|Texas Instruments Incorporated
|Reference-Less PCIe Gen 1-6 Compliant Programmable BAW Clock Generator
| Marketing Part # : LMK3H210X
| Digital Voltage Range : 1.8V, 2.5V, 3.3V
| Package-type: RER
| #pins/pkg drawing : 40/24-pin VQFN
[IBIS Ver] 4.1
[File name] lmk3h210x.ibs
[File Rev] 1.0
[Date] 06/26/2025
[Source]
| Texas Instruments Incorporated.
| 12500 TI Blvd
| Dallas, TX -75243
[Notes] Revision History:
| Rev 1.0: 6/26/2025
| - Initial version of the model
| - Model generated from simulations in TISPICE/SPECTRE
| - C_comp although listed in numerical order of value are
| obtained from varying PVT conditions. For PVT conditions for
| each specific value refer the buffer description under
| respective [Model]. IBIS model user is responsible for using
| appropriate C_comp to simulate for Signal Integrity.
| - Warnings regarding combined Non-monotonicity of various models have been
| reviewed and considered minor and can be ignored.
|**** Modify the following if you use [Model Selector]*****************
| - Model names with a trailing _1p8 contain the model for
| 1.8V operation. Model names with a trailing _3p3 contain the model
| for 3.3V operation.
[Disclaimer]
| This model is designed as an aid for customers of Texas Instruments.
| TI and its licensors and suppliers make no warranties, either expressed
| or implied, with respect to this model, including the warranties of
| merchantability or fitness for a particular purpose. The model is
| provided solely on an "as is" basis. The entire risk as to its quality
| and performance is with the customer.
| This model is subject to change without notice. Texas Instruments
| Incorporated is not responsible for updating this model.
[Copyright]
(C) Copyright 2023 Texas Instruments Incorporated. All rights reserved.
[Component] LMK3H2108
[Manufacturer] Texas Instruments Incorporated
[Package] |RKP (VQFN) 40-pin
| variable typ min max
R_pkg 0.05 0.04 0.06
L_pkg 1.0nH 0.8nH 1.2nH
C_pkg 0.2pF 0.16pF 0.24pF
| pin number (pin name) mapping to model name
[Pin] signal_name model_name R_pin L_pin C_pin
1	IN0_P	input	0.12641	1.67082n	0.21025p
2	IN0_N	input	0.11581	1.486n	0.20759p
3	VDDX	power	0.10567	1.34427n	0.19938p
4	IN1_P	input	0.10345	1.29467n	0.19198p
5	IN1_N	input	0.10152	1.28238n	0.18846p
6	VDDR	power	0.10149	1.27988n	0.18625p
7	IN2_P	input	0.10331	1.2926n	0.19439p
8	IN2_N	input	0.10916	1.38037n	0.19925p
9	SCL	scl	0.1192	1.5418n	0.21165p
10	SDA	sda	0.13133	1.74296n	0.21079p
11	VDDD	power	0.06193	1.26238n	0.24131p
12	GPIO_0	gpi	0.11504	1.47538n	0.20933p
13	GPIO_1	gpi	0.11121	1.42355n	0.20184p
14	GPIO_2	oe	0.10542	1.32585n	0.1916p
15	GPIO_3	oe	0.10179	1.28213n	0.18774p
16	GPIO_4	gpo	0.10307	1.29989n	0.19177p
17	NC	nc	NA	NA	NA
18	VDDO_0	power	0.11559	1.49016n	0.20467p
19	OUT0_N	output	0.12902	1.69101n	0.22272p
20	OUT0_P	output	0.14193	1.91736n	0.22281p
21	VDDO1_2	power	0.12064	1.57469n	0.19586p
22	OUT1_N	output	0.11031	1.41063n	0.20163p
23	OUT1_P	output	0.10413	1.30684n	0.19475p
24	OUT2_N	output	0.10253	1.28873n	0.19329p
25	OUT2_P	output	0.10215	1.28641n	0.18943p
26	OUT3_N	output	0.10306	1.29805n	0.18796p
27	OUT3_P	output	0.10956	1.38812n	0.19942p
28	OUT4_N	output	0.11218	1.43239n	0.20389p
29	OUT4_P	output	0.12463	1.61491n	0.21636p
30	VDDO3_4	power	0.13578	1.81915n	0.21363p
31	OUT5_N	output	0.12381	1.62136n	0.19949p
32	OUT5_P	output	0.11279	1.44821n	0.20437p
33	VDDO_5	power	0.10527	1.32351n	0.19485p
34	VDDO_6	power	0.10149	1.2793n	0.19123p
35	OUT6_N	output	0.10439	1.31083n	0.19125p
36	OUT6_P	output	0.11058	1.41183n	0.1996p
37	OUT7_N	output	0.11354	1.45518n	0.20444p
38	OUT7_P	output	0.12617	1.64272n	0.21886p
39	VDDO_7	power	0.14093	1.87977n	0.23888p
40	VDDA	power	0.15681	2.13658n	0.24857p
| Differential pin definition
| Use in differential output types, LP-HCSL, LVDS
[Diff Pin] inv_pin vdiff tdelay_typ tdelay_min tdelay_max
| The 'OUTx_P' pin is Diff_pin and the 'OUTx_N' pin is the inv_pin|
1	2	10m	NA	NA	NA
4	5	10m	NA	NA	NA
7	8	10m	NA	NA	NA
19	20	NA	NA	NA	NA
22	23	NA	NA	NA	NA
24	25	NA	NA	NA	NA
26	27	NA	NA	NA	NA
28	29	NA	NA	NA	NA
31	32	NA	NA	NA	NA
35	36	NA	NA	NA	NA
37	38	NA	NA	NA	NA
[Series Pin Mapping] pin_2 model_name function_table_group
|1	2	 rterm_lvds_100  | Uncomment to instantiate LVDS Termination
|4	5	 rterm_lvds_100  | Uncomment to instantiate LVDS Termination
|7	8	 rterm_lvds_100  | Uncomment to instantiate LVDS Termination
[Component] LMK3H2104
[Manufacturer] Texas Instruments Incorporated
[Package] |RKP (VQFN) 24-pin
| variable typ min max
R_pkg 0.05 0.04 0.06
L_pkg 1.0nH 0.8nH 1.2nH
C_pkg 0.2pF 0.16pF 0.24pF
| pin number (pin name) mapping to model name
[Pin] signal_name model_name R_pin L_pin C_pin
1	IN0_P	input	0.08053	0.95214n	0.14352p
2	IN0_N	input	0.07028	0.8079n	0.14775p
3	REF_1	ref_out	0.07263	0.83964n	0.14937p
4	SCL	scl	0.07571	0.88875n	0.15057p
5	SDA	sda	0.07012	0.80851n	0.1479p
6	GPI_2	gpi	0.08007	0.9478n	0.14072p
7	VDDO	power	0.0388	0.64762n	0.16177p
8	GPIO_0	oe	0.07015	0.80671n	0.14886p
9	GPIO_1	gpo	0.07269	0.84224n	0.15183p
10	OUT0_N	output	0.07104	0.81871n	0.14663p
11	OUT0_P	output	0.07328	0.85018n	0.15073p
12	VDDO_0	power	0.08936	1.08497n	0.14963p
13	OUT1_N	output	0.07771	0.9126n	0.51008p
14	OUT1_P	output	0.07026	0.80586n	0.5238p
15	VDDO_1	power	0.07074	0.81241n	0.519p
16	OUT2_N	output	0.07163	0.82615n	0.52562p
17	OUT2_P	output	0.07416	0.8615n	0.5263p
18	VDDO_2	power	0.08732	1.0469n	0.51975p
19	OUT3_P	output	0.07624	0.89807n	0.5098p
20	OUT3_N	output	0.07024	0.80339n	0.52367p
21	VDDO_3	power	0.03808	0.62617n	0.17515p
22	VDDA	power	0.03507	0.55683n	0.17375p
23	REF_0	ref_out	0.07052	0.81036n	0.15464p
24	VDD_REF	power	0.03929	0.64651n	0.16417p
| Differential pin definition
| Use in differential output types, LP-HCSL, LVDS
[Diff Pin] inv_pin vdiff tdelay_typ tdelay_min tdelay_max
| The 'OUTx_P' pin is Diff_pin and the 'OUTx_N' pin is the inv_pin|
1	2	10m	NA	NA	NA
10	11	NA	NA	NA	NA
13	14	NA	NA	NA	NA
16	17	NA	NA	NA	NA
19	20	NA	NA	NA	NA
[Series Pin Mapping] pin_2 model_name function_table_group
|1	2	 rterm_lvds_100 | Uncomment to instantiate LVDS Termination
| Model Selectors
[Model Selector] output
LPHCSL_100 LP-HCSL with 100O output termination
LPHCSL_85 LP-HCSL with 85O output termination
CMOS_1P8V_FSLEW CMOS with 1.8V VDD and Fast Slew rate
CMOS_1P8V_SSLEW CMOS with 1.8V VDD and Slow Slew rate
CMOS_2P5V_FSLEW CMOS with 2.5V VDD and Fast Slew rate
CMOS_2P5V_SSLEW CMOS with 2.5V VDD and Slow Slew rate
CMOS_3P3V_FSLEW CMOS with 3.3V VDD and Fast Slew rate
CMOS_3P3V_SSLEW CMOS with 3.3V VDD and Slow Slew rate
CMOS1P2_VDD18 1.2V CMOS with 1.8V VDD
CMOS1P2_VDD25 1.2V CMOS with 2.5V VDD
CMOS1P2_VDD33 1.2V CMOS with 3.3V VDD
LVDS_1P8 LVDS with 1.8V VDD
LVDS_2P5 LVDS with 2.5V VDD
LVDS_3P3 LVDS with 3.3V VDD
[Model Selector] input
CKINPUT_NOTERM_1P8V No termination, 1.8V VDD
CKINPUT_WBIAS_1P8V No termination, Internal bias enabled, 1.8V VDD
CKINPUT_50GND_1P8V 50ohm to ground termination, 1.8V VDD
CKINPUT_NOTERM_2P5V No termination, 2.5V VDD
CKINPUT_WBIAS_2P5V No termination, Internal bias enabled, 2.5V VDD
CKINPUT_50GND_2P5V 50ohm to ground termination, 2.5V VDD
CKINPUT_NOTERM_3P3V No termination, 3.3V VDD
CKINPUT_WBIAS_3P3V No termination, Internal bias enabled, 3.3V VDD
CKINPUT_50GND_3P3V 50ohm to ground termination, 3.3V VDD
CKINPUT_CMOS	CMOS Input RX
[Model Selector] ref_out
REF_CLK_1P8 CMOS REF_OUT with 1.8V VDD
REF_CLK_2P5 CMOS REF_OUT with 2.5V VDD
REF_CLK_3P3 CMOS REF_OUT with 3.3V VDD
INPUT_CTRL_1P8 ctrl input with 1.8V VDD
INPUT_CTRL_2P5 ctrl input with 2.5V VDD
INPUT_CTRL_3P3 ctrl input with 3.3V VDD
[Model Selector] oe
INPUT_LS_OE_PD_1P8 OE input with 75k pulldown with 1.8V VDD
INPUT_LS_OE_PD_2P5 OE input with 75k pulldown with 2.5V VDD
INPUT_LS_OE_PD_3P3 OE input with 75k pulldown with 3.3V VDD
INPUT_LS_OE_PU_1P8 OE input with 75k pullup with 1.8V VDD
INPUT_LS_OE_PU_2P5 OE input with 75k pullup with 2.5V VDD
INPUT_LS_OE_PU_3P3 OE input with 75k pullup with 3.3V VDD
[Model Selector] gpi
GPI_weakPD_1P8 general purpose input with weak pulldown with 1.8V VDD
GPI_weakPD_2P5 general purpose input with weak pulldown with 2.5V VDD
GPI_weakPD_3P3 general purpose input with weak pulldown with 3.3V VDD
GPI_HS_OE_PD_1P8 second OE with 75k pulldown with 1.8V VDD
GPI_HS_OE_PD_2P5 second OE with 75k pulldown with 2.5V VDD
GPI_HS_OE_PD_3P3 second OE with 75k pulldown with 3.3V VDD
[Model Selector] gpo
GPIO_CMOS1P8V GPO with CMOS 1.8V
GPIO_CMOS2P5V GPO with CMOS 2.5V
GPIO_CMOS3P3V GPO with CMOS 3.3V
[Model Selector] scl
INPUT_I2C_1P8 SCL input with 1.8V VDD
INPUT_I2C_2P5 SCL input with 2.5V VDD
INPUT_I2C_3P3 SCL input with 3.3V VDD
[Model Selector] sda
OUTPUT_I2C_1P8 SDA output  with 1.8V VDD
OUTPUT_I2C_2P5 SDA output  with 2.5V VDD
OUTPUT_I2C_3P3 SDA output  with 3.3V VDD
INPUT_I2C_1P8 I2C input with 1.8V VDD
INPUT_I2C_2P5 I2C input with 2.5V VDD
INPUT_I2C_3P3 I2C input with 3.3V VDD
[Model] rterm_lvds_100
Model_type Series
C_comp 0.0000pF 0.0000pF 0.0000pF
[Temperature Range]   45   125   -40
[Voltage Range]   3.3   2.97V   3.597V
[R Series]   100   125   75
| Models and submodels in the file (52): rterm_lvds_100 (Series), CKINPUT_WBIAS_3P3V (Input), CKINPUT_NOTERM_3P3V (Input), CKINPUT_50GND_3P3V (Input), CKINPUT_WBIAS_2P5V (Input), CKINPUT_NOTERM_2P5V (Input), CKINPUT_50GND_2P5V (Input), CKINPUT_NOTERM_1P8V (Input), CKINPUT_WBIAS_1P8V (Input), CKINPUT_50GND_1P8V (Input), CKINPUT_CMOS (Input), LPHCSL_100 (Output), LPHCSL_85 (Output), CMOS1P2_VDD18 (Output), CMOS1P2_VDD25 (Output), CMOS1P2_VDD33 (Output), CMOS_1P8V_FSLEW (Output), CMOS_1P8V_SSLEW (Output), CMOS_2P5V_FSLEW (Output), CMOS_2P5V_SSLEW (Output), CMOS_3P3V_FSLEW (Output), CMOS_3P3V_SSLEW (Output), LVDS_1P8 (Output), LVDS_2P5 (Output), LVDS_3P3 (Output), REF_CLK_1P8 (Output), REF_CLK_2P5 (Output), REF_CLK_3P3 (Output), INPUT_I2C_1P8 (Input), INPUT_I2C_2P5 (Input), INPUT_I2C_3P3 (Input), OUTPUT_I2C_1P8 (Open_drain), OUTPUT_I2C_2P5 (Open_drain), OUTPUT_I2C_3P3 (Open_drain), INPUT_CTRL_1P8 (Input), INPUT_CTRL_2P5 (Input), INPUT_CTRL_3P3 (Input), INPUT_LS_OE_PD_1P8 (Input), INPUT_LS_OE_PD_2P5 (Input), INPUT_LS_OE_PD_3P3 (Input), INPUT_LS_OE_PU_1P8 (Input), INPUT_LS_OE_PU_2P5 (Input), INPUT_LS_OE_PU_3P3 (Input), GPI_HS_OE_PD_1P8 (Input), GPI_HS_OE_PD_2P5 (Input), GPI_HS_OE_PD_3P3 (Input), GPI_weakPD_1P8 (Input), GPI_weakPD_2P5 (Input), GPI_weakPD_3P3 (Input), GPIO_CMOS1P8V (Output), GPIO_CMOS2P5V (Output), GPIO_CMOS3P3V (Output)
